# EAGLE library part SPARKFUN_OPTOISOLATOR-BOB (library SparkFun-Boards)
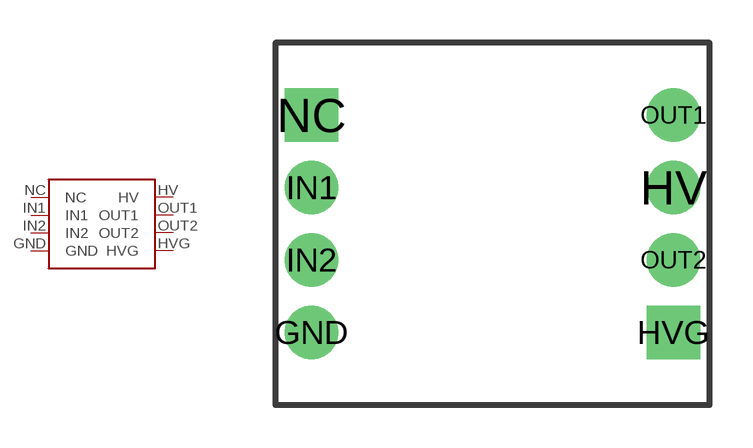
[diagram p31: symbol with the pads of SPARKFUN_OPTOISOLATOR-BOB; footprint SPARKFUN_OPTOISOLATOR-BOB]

Designator prefix -

## SPARKFUN_OPTOISOLATOR-BOB  [SPARKFUN_OPTOISOLATOR-BOB]
GND  GND
HV  HV
HVG  HVG
IN1  IN1
IN2  IN2
NC  NC
OUT1  OUT1
OUT2  OUT2

## Footprint SPARKFUN_OPTOISOLATOR-BOB (pad centres in mm)
drill 1.016 pad 1.88: GND -6.35,-3.81; HV 6.35,1.27; IN1 -6.35,1.27; IN2 -6.35,-1.27; OUT1 6.35,3.81; OUT2 6.35,-1.27
drill 1.016 pad 1.88 square: HVG 6.35,-3.81; NC -6.35,3.81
